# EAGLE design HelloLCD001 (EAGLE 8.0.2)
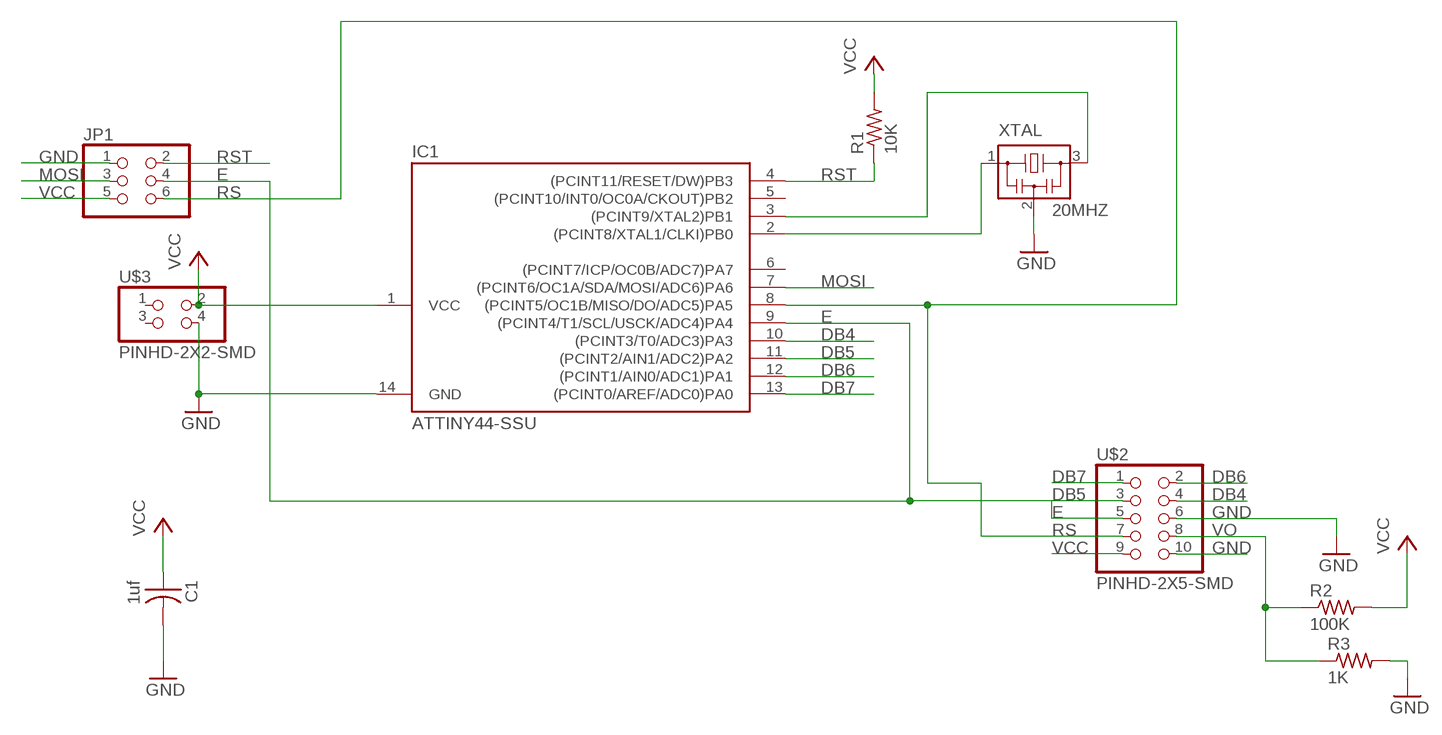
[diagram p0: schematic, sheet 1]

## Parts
C1  1uf  CAP-US1206FAB  [C1206FAB]
IC1  ATTINY44-SSU  [SOIC14]
JP1  PINHD-2X3-SMD  [2X03SMD]
R1  10K  RES-US1206FAB  [R1206FAB]
R2  100K  RES-US1206FAB  [R1206FAB]
R3  1K  RES-US1206FAB  [R1206FAB]
U$2  PINHD-2X5-SMD  [2X05SMD]
U$3  PINHD-2X2-SMD  [2X02SMD]
XTAL  20MHZ  RESONATOR  [EFOBM]

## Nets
DB4: IC1.10((PCINT3/T0/ADC3)PA3) U$2.4
DB5: IC1.11((PCINT2/AIN1/ADC2)PA2) U$2.3
DB6: IC1.12((PCINT1/AIN0/ADC1)PA1) U$2.2
DB7: IC1.13((PCINT0/AREF/ADC0)PA0) U$2.1
E: IC1.9((PCINT4/T1/SCL/USCK/ADC4)PA4) JP1.4 U$2.5
GND: C1.2 IC1.14(GND) JP1.1 R3.2 U$2.6 U$2.10 U$3.4 XTAL.2
MOSI: IC1.7((PCINT6/OC1A/SDA/MOSI/ADC6)PA6) JP1.3
N$2: IC1.3((PCINT9/XTAL2)PB1) XTAL.3
N$3: IC1.2((PCINT8/XTAL1/CLKI)PB0) XTAL.1
RS: IC1.8((PCINT5/OC1B/MISO/DO/ADC5)PA5) JP1.6 U$2.7
RST: IC1.4((PCINT11/RESET/DW)PB3) JP1.2 R1.1
VCC: C1.1 IC1.1(VCC) JP1.5 R1.2 R2.2 U$2.9 U$3.2
VO: R2.1 R3.1 U$2.8
Unconnected: IC1.5((PCINT10/INT0/OC0A/CKOUT)PB2) IC1.6((PCINT7/ICP/OC0B/ADC7)PA7) U$3.1 U$3.3

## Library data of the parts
C1 = fab:CAP-US
IC1 = fab:ATTINY44
JP1 = fab:PINHD-2X3-SMD: PIN HEADER
R1-R3 = fab:RES-US: Resistor (US Symbol)
U$2 = fab:PINHD-2X5-SMD
U$3 = fab:PINHD-2X2-SMD
XTAL = fab:RESONATOR

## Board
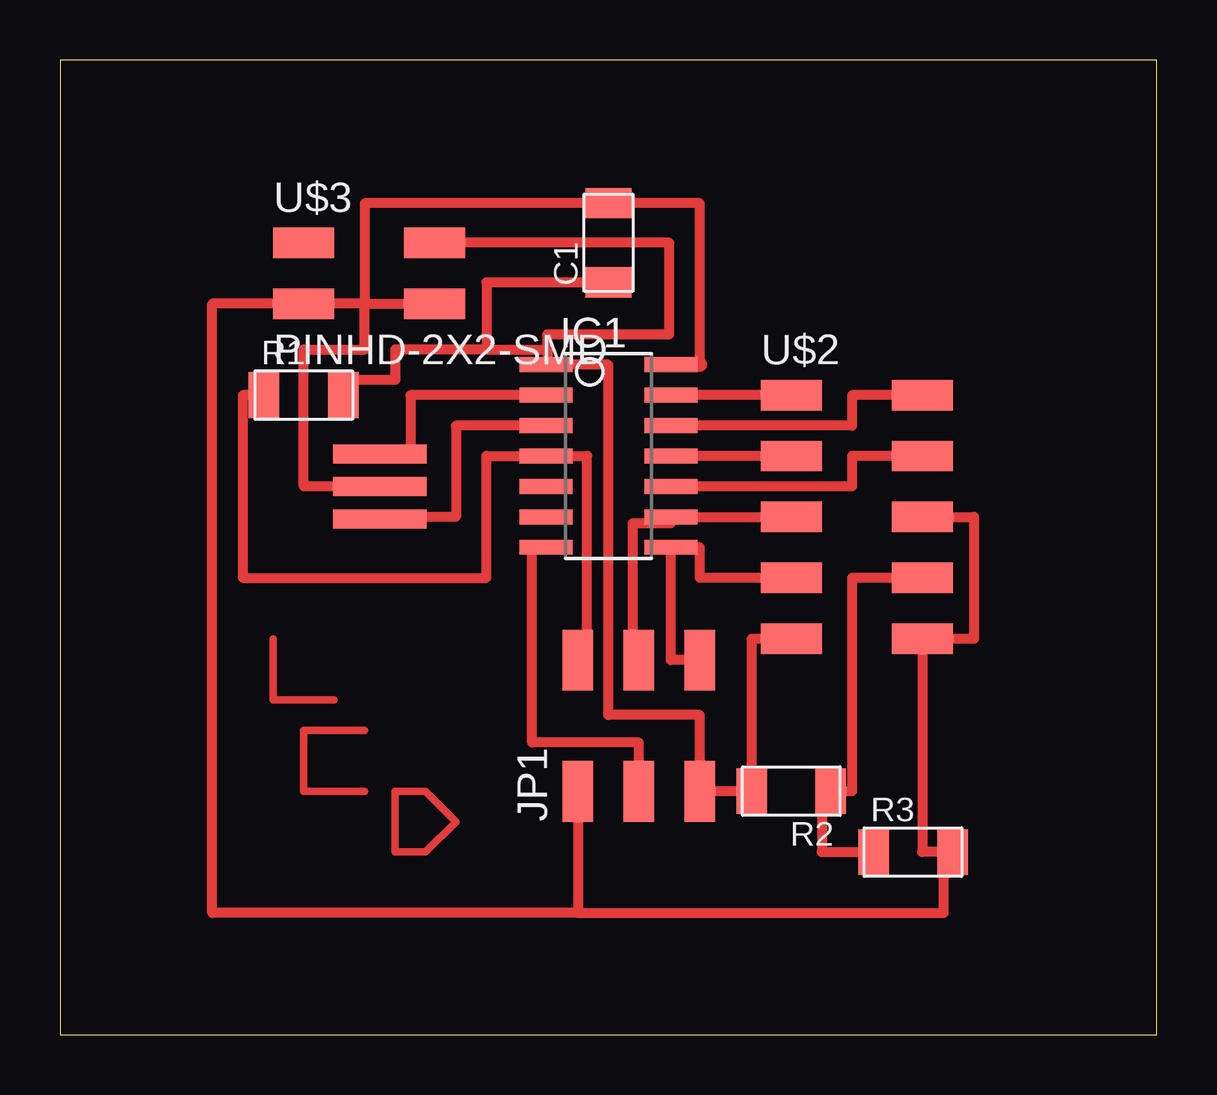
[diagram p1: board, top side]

Size 45.72 x 40.64 mm. Coordinates in mm from the lower left corner, seen from the top.
Outline: 0,0 45.72,0 45.72,40.64 0,40.64 0,0
Copper layers (1*16): Top 0.035mm / dielectric 1.5mm / Bottom 0.035mm
Design rules "default": minimum track width 10mil, minimum drill 24mil, track to track 8mil, track to pad 8mil, pad to pad 8mil, via to via 8mil, smd to smd 8mil, copper to edge 40mil, drill to drill 8mil, minimum pad ring 10mil, minimum via ring 8mil, stop-mask expansion 4mil, vias tented up to drill 0mil, thermal gap 10mil

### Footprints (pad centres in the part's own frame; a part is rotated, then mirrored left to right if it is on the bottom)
C1206FAB = smd 1.27 x 1.905: 1 -1.651,0; 2 1.651,0
SOIC14 = smd 0.61 x 2.21: 1 -3.81,-2.603; 2 -2.54,-2.603; 3 -1.27,-2.603; 4 0,-2.603; 5 1.27,-2.603; 6 2.54,-2.603; 7 3.81,-2.603; 8 3.81,2.603; 9 2.54,2.603; 10 1.27,2.603; 11 0,2.603; 12 -1.27,2.603; 13 -2.54,2.603; 14 -3.81,2.603
2X03SMD = smd 2.54 x 1.27: 1 -2.54,2.54; 2 2.92,2.54; 3 -2.54,0; 4 2.92,0; 5 -2.54,-2.54; 6 2.92,-2.54
R1206FAB = smd 1.27 x 1.905: 1 -1.651,0; 2 1.651,0
2X05SMD = smd 2.54 x 1.27: 1 -2.54,2.54; 2 2.92,2.54; 3 -2.54,0; 4 2.92,0; 5 -2.54,-2.54; 6 2.92,-2.54; 7 -2.54,-5.08; 8 2.92,-5.08; 9 -2.54,-7.62; 10 2.92,-7.62
2X02SMD = smd 2.54 x 1.27: 1 -2.54,1.27; 2 2.92,1.27; 3 -2.54,-1.27; 4 2.92,-1.27
EFOBM = smd 0.8 x 3.9: 1 -1.35,0; 2 0,0; 3 1.35,0

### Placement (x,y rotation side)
C1  22.86,33.02 90 top
IC1  22.86,24.13 270 top
JP1  24.13,12.7 90 top
R1  10.16,26.67 0 top
R2  30.48,10.16 180 top
R3  35.56,7.62 0 top
U$2  33.02,24.13 0 top
U$3  12.7,31.75 0 top
XTAL  13.34,22.86 270 top

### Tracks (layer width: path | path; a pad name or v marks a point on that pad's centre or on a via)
DB4
  Top 0.406: U$2.4 33.02,24.13 33.02,22.86 IC1.10
DB5
  Top 0.406: U$2.3 IC1.11
DB6
  Top 0.406: IC1.12 33.02,25.4 33.02,26.67 U$2.2
DB7
  Top 0.406: U$2.1 IC1.13
E
  Top 0.406: U$2.5 IC1.9 25.46,21.34 23.88,21.34 23.88,16.26 24.13,16.26 JP1.4
GND
  Top 0.406: 21.59,5.08 36.83,5.08 36.83,7.62 R3.2 35.94,7.62 U$2.10 38.1,16.51 38.1,21.59 U$2.6 | 21.59,5.08 6.35,5.08 6.35,30.48 12.7,30.48 | 26.67,27.94 26.67,34.67 C1.2 12.7,34.67 12.7,30.48 | 12.7,30.48 U$3.4 | XTAL.2 10.16,22.86 10.16,28.57 12.7,28.57 12.7,30.48 | JP1.1 21.59,5.08
  Top 0.61: IC1.14 26.67,27.94
MOSI
  Top 0.406: IC1.7 19.68,20.32 19.68,12.19 24.13,12.19 JP1.3
N$1
  Top 0.305: 8.89,16.51 8.89,13.97 11.43,13.97
N$2
  Top 0.406: XTAL.3 12.7,21.59 16.51,21.59 16.51,25.4 IC1.3
N$3
  Top 0.406: IC1.2 14.61,26.67 14.61,24.13 12.7,24.13 XTAL.1
N$4
  Top 0.305: 12.7,12.7 10.16,12.7 10.16,10.16 12.7,10.16
N$5
  Top 0.305: 13.97,8.89 13.97,7.62 15.24,7.62 16.51,8.89 15.24,10.16 13.97,10.16 13.97,8.89
RS
  Top 0.406: U$2.7 26.67,19.05 26.67,20.32 IC1.8 25.46,15.62 JP1.6
RST
  Top 0.406: JP1.2 21.97,15.62 21.97,24.13 IC1.4 17.78,24.13 17.78,19.05 7.62,19.05 7.62,26.67 R1.1
VCC
  Top 0.406: U$2.9 28.83,16.51 R2.2 JP1.5 26.67,13.34 22.86,13.34 22.86,27.94 IC1.1 20.32,27.94 20.32,28.57 | C1.1 17.78,31.37 17.78,28.57 | 17.78,28.57 13.97,28.57 13.97,27.3 11.81,27.3 R1.2 | U$3.2 25.4,33.02 25.4,29.21 20.32,29.21 20.32,28.57 | 17.78,28.57 20.32,28.57
VO
  Top 0.406: R3.1 31.75,7.62 31.75,10.16 R2.1 33.02,10.16 33.02,19.05 U$2.8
